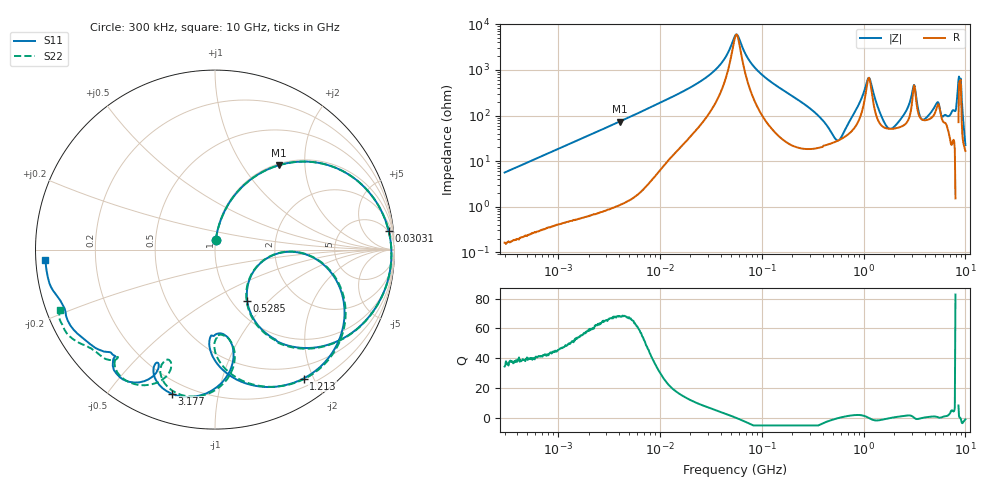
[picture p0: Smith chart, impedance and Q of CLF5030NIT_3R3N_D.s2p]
! S-Parameter Data Generated by TDK Corporation
! Copyright(C) 2019 TDK Corporation.
! All Rights Reserved.
! TDK P/N: CLF5030NIT-3R3N-D (Inductor)
! Property: L=3.3uH at 100kHz
! Size(LxWxT): 5.3x5x2.7mm
! Model Type: s2p (Touchstone File Format Version 1.0)
! Frequency: DC=Yes Start=0.3MHz Stop=10000MHz 802points Log-sweep
! Model Generated on May 10, 2019
! Port Assignments:
!  1 ---@@@--- 2
! Applicable Conditions:
!  Temperature = 25 degC
!  DC Bias Current = 0 A
!  Small Signal Operation
! Terms and conditions regarding TDK Simulation Models
! (1)This simulation model is being provided solely for informational purposes. Please refer to the specifications of the products in terms of detailed characteristics of such products.
! (2)In no event shall TDK Corporation of any of its subsidiaries be liable for any loss or damage arising, directly or indirectly,
!  From any information contained in this simulation model, including, but not limited to loss or damages arising from any inaccuracies, omissions or errors in connection with such information.
! (3)Any and all copyrights on this simulation model are owned by TDK Corporation.
!  Duplication or redistribution of this simulation model without prior written permission from TDK Corporation is prohibited.
! (4)This simulation model is subject to any modification or change without any prior notice.
! (5)Neither TDK Corporation nor any of its subsidiaries shall make any warranty, express or implied,
!  Including but not limited to the correctness, implied warranties of merchantability and fitness for a particular purpose with respect to this simulation models.
! (6)The use of this simulation model shall be deemed to have consented to the terms and conditions hereof.
# Hz S MA R 50
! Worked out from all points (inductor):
!   801 points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, 300 kHz to 10 GHz, reference 50 ohm
!   read as one part in series: L = 2.96 uH near 318.3 kHz
!   highest Q = 68.2 at 4.054 MHz (marker M1), where L = 2.9 uH
!   self-resonance near 56.34 MHz
!   S11 on the Smith chart (normalised r, x): 300 kHz: 1.00, +0.11; 30.31 MHz: 4, +18; 528.5 MHz: 1.17, -0.76; 1.213 GHz: 0.31, -1.86; 3.177 GHz: 0.14, -0.73; 10 GHz: 0.03, -0.03
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300000  0.05617 85.2  0.9968 -3.2  0.9965 -3.2  0.05618 85.4
1713600  0.2962 71.7  0.9498 -17.3  0.9498 -17.3  0.2962 71.7
4053600  0.5892 52.9  0.7993 -36.2  0.7994 -36.2  0.5893 52.9
9671944  0.8646 28.0  0.4762 -60.2  0.4762 -60.2  0.8646 28.0
3.031424e7  0.9733 6.1  0.1287 -75.6  0.1287 -75.6  0.9733 6.1
5.477226e7  0.9835 -1.8  0.01764 -23.0  0.01765 -23.0  0.9835 -1.9
1.050124e8  0.9751 -11.8  0.1337 71.2  0.1338 71.2  0.9751 -12.0
3.126428e8  0.776 -44.7  0.5382 37.6  0.5383 37.6  0.7758 -45.2
5.285151e8  0.3372 -57.9  0.7545 -5.7  0.7547 -5.7  0.335 -58.3
6.242396e8  0.2491 -25.2  0.7468 -24.9  0.747 -24.9  0.2475 -25.0
7.84152e8  0.5034 -2.9  0.6002 -54.9  0.6004 -54.9  0.5066 -2.8
9.903836e8  0.807 -26.6  0.2713 -81.0  0.2715 -81.0  0.8126 -26.4
1.212691e9  0.8714 -55.5  0.1653 -5.6  0.1654 -5.7  0.8766 -54.9
1.767019e9  0.5644 -92.6  0.5107 -42.6  0.5108 -42.6  0.5691 -89.9
2.53795e9  0.5899 -79.9  0.3885 -111.4  0.3886 -111.4  0.6327 -80.2
3.177248e9  0.8385 -106.8  0.06726 -85.8  0.06711 -86.5  0.8105 -108.8
3.932853e9  0.7063 -116.7  0.2807 -93.3  0.2806 -93.3  0.6656 -112.7
5.284132e9  0.887 -125.4  0.1036 -145.1  0.1035 -145.1  0.8799 -122.7
6.656819e9  0.8309 -136.7  0.1233 -172.0  0.1235 -172.0  0.8721 -138.4
7.763894e9  0.9101 -152.4  0.04672 147.6  0.0467 147.4  0.9436 -149.3
8.881947e9  0.924 -164.8  0.004179 -141.2  0.00382 -142.5  0.9212 -158.2
1e10  0.9464 -176.6  0.0309 -70.5  0.03092 -71.2  0.9275 -158.8
